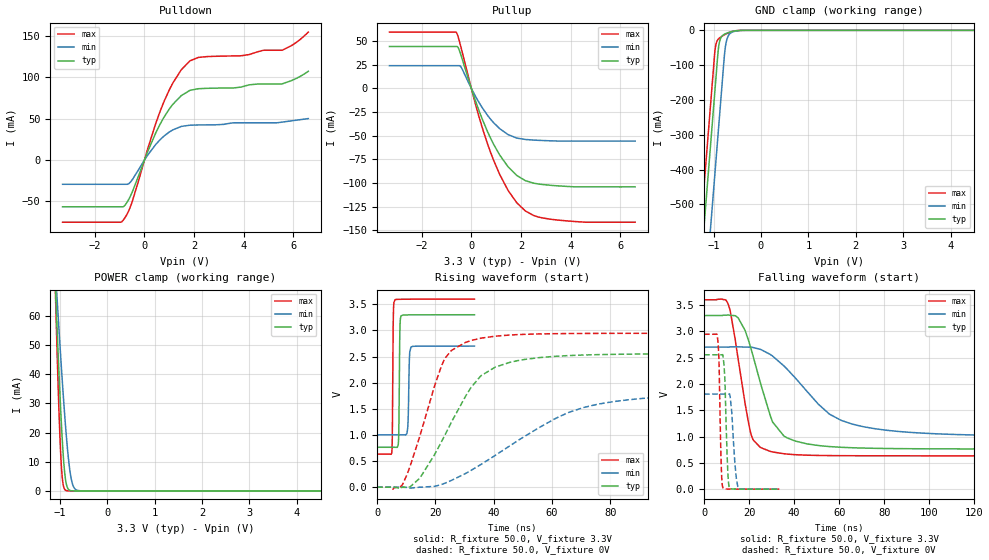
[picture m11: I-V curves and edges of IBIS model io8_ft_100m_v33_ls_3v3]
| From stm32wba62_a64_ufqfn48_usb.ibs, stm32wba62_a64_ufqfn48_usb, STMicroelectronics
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[Model]   io8_ft_100m_v33_ls_3v3
Model_type I/O
Polarity   Non-Inverting
Enable   Active-Low
| CAP_THRESHOLD on pad IOFT is "UDTCAPC" :
| Rising=30.0% of vddiom   Falling=70.0% of vddiom
| C_comp min and max val. don't necessarily correlate with the min and max pvt
| but are the smallest and greatest pad capacitance found.
| var   typ   min   max
C_comp   3.88673pF  3.77800pF  3.94187pF
|C_comp_pullup   2.41834pF  2.25933pF  2.53603pF
|C_comp_pulldown   1.46839pF  1.51868pF  1.40584pF
Vinl = 1.35V
Vinh = 1.8V
Vmeas = 1.65V   | Reference voltage for timing measurements
Cref  = 50.0pF   | Timing specification test load capacitance value
Rref  = 1.0MOhm   | Timing specification test load resistance value
Vref  = 1.815V   | Timing specification test load voltage
[Model Spec]
| TIME_THRESHOLD on pin ZIV33M is "CMOS" :
| Rising=50.0% of vddiom   Falling=50.0% of vddiom
Vinl 1.28450V 1.07450V 1.37050V
Vinh 1.79550V 1.51850V 1.89950V
| variable   typ   min   max
[Temperature Range] 25.0 140.0 -40.0
| variable   typ   min   max
[Voltage Range] 3.3V 2.7V 3.6V
| variable   typ   min   max
[POWER Clamp Reference] 3.3V 2.7V 3.6V
| variable   typ   min   max
[GND Clamp Reference] 0V 0V 0V
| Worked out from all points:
|   slope of the pulldown table from 0 to 0.495 V, typ, clamps not added: 14 ohm
|   slope of the pullup table from 0 to 0.495 V, typ, clamps not added: 13.8 ohm
|   GND clamp passes 1 mA (typ) near -0.51 V on its own axis
|   POWER clamp passes 1 mA (typ) near -0.83 V on its own axis
|   rising waveform, R_fixture 50.0, V_fixture 3.3V: 20-80 % time 263ps typ, 359ps min, 246ps max; typ from 0.764 V to 3.3 V
|   falling waveform, R_fixture 50.0, V_fixture 3.3V: 20-80 % time 10.6ns typ, 24.4ns min, 6.74ns max; typ from 3.3 V to 0.764 V
|   rising waveform, R_fixture 50.0, V_fixture 0V: 20-80 % time 15.8ns typ, 33.1ns min, 9.96ns max; typ from 0 V to 2.55 V
|   falling waveform, R_fixture 50.0, V_fixture 0V: 20-80 % time 1.09ns typ, 1.66ns min, 865ps max; typ from 2.55 V to 0 V
[POWER Clamp]
-3.3V     1.123A     753mA      1.645A
-1.09V    69.42mA    75.17mA    67.14mA
-1.08V    65.31mA    72.42mA    61.23mA
-1.06V    57.23mA    66.98mA    49.77mA
-1.01V    38.06mA    53.68mA    24.29mA
-970mV    24.36mA    43.46mA    9.575mA
-930mV    13.06mA    33.74mA    2.352mA
-870mV    3.065mA    20.56mA    165.9uA
-810mV    418.4uA    10.06mA    10.3uA
-760mV    69.41uA    4.321mA    1.009uA
-630mV    611.5nA    197uA      2.727nA
6.6V      0A         0A         0A
[GND Clamp]
-3.3V     -4.134A    -4.372A    -4.018A
-1.59V    -1.227A    -1.465A    -1.111A
-1.25V    -648.9mA   -886.9mA   -533mA
-980mV    -189.9mA   -427.9mA   -74mA
-960mV    -155.9mA   -393.9mA   -48.8mA
-910mV    -70.86mA   -308.9mA   -27.2mA
-880mV    -37.23mA   -257.9mA   -22.76mA
-770mV    -11.28mA   -71.59mA   -12.95mA
-730mV    -8.709mA   -32.74mA   -10.07mA
-630mV    -4.122mA   -6.943mA   -4.354mA
-370mV    -42.68uA   -212.2uA   -13.03uA
6.6V      2.31nA     506.4nA    1.057nA
| variable   typ   min   max
[Pullup Reference] 3.3V 2.7V 3.6V
| variable   typ   min   max
[Pulldown Reference] 0V 0V 0V
[Pullup]
-3.3V     44.29mA    24.03mA    59.52mA
-600mV    44.29mA    24.03mA    58.97mA
-520mV    42.47mA    24.03mA    53.36mA
-410mV    34.41mA    22.34mA    42.54mA
310mV     -23.64mA   -14.94mA   -30.17mA
890mV     -58.72mA   -36.07mA   -75.54mA
1.48V     -82.86mA   -48.82mA   -107.8mA
1.83V     -91.99mA   -52.47mA   -120.8mA
2.17V     -97.42mA   -53.93mA   -129.4mA
2.7V      -101mA     -54.85mA   -135.9mA
3.48V     -102.9mA   -55.62mA   -139.1mA
6.6V      -104.1mA   -55.62mA   -141.4mA
[Pulldown]
-3.3V     -56.7mA    -29.42mA   -75.36mA
-860mV    -56.67mA   -29.42mA   -72.94mA
-520mV    -40.69mA   -25.01mA   -52.64mA
460mV     33.25mA    19.09mA    44.92mA
800mV     52.54mA    29.36mA    71.75mA
1.14V     67.41mA    36.49mA    93.2mA
1.48V     77.97mA    40.67mA    109.3mA
1.83V     84.38mA    42.18mA    120.1mA
2.17V     86.37mA    42.45mA    124.3mA
3.88V     88.31mA    45.11mA    126.3mA
5.54V     92.28mA    45.89mA    133mA
6.6V      107.5mA    50.2mA     155mA
[Ramp]
dV/dt_r 1.53258V/15.4843ns 1.08428V/32.98714ns 1.76673V/9.86055ns
dV/dt_f 1.52157V/10.47685ns 1.01877V/24.02377ns 1.77971V/6.67032ns
R_load = 50.0
| Removed startup time: 0s 0s 0s  .
| Removed end time: 33.4ns.
[Rising Waveform]
R_fixture   = 50.0
V_fixture   = 3.3V
V_fixture_min = 2.7V
V_fixture_max = 3.6V
0s        764mV      1.002V     633.8mV
5ns       764.1mV    1.002V     653.2mV
5.55ns    764.1mV    1.002V     3.255V
6.15ns    764.1mV    1.002V     3.589V
7.35ns    913.7mV    1.002V     3.595V
7.8ns     2.993V     1.002V     3.595V
8.2ns     3.278V     1.002V     3.596V
10.5ns    3.297V     1.142V     3.597V
11.6ns    3.298V     2.684V     3.597V
33.4ns    3.3V       2.699V     3.6V
| Removed startup time: 0s 0s 0s  .
| Removed end time: 248.4ns.
[Falling Waveform]
R_fixture   = 50.0
V_fixture   = 3.3V
V_fixture_min = 2.7V
V_fixture_max = 3.6V
0s        3.3V       2.7V       3.6V
10.55ns   3.31V      2.7V       3.534V
11.75ns   3.303V     2.706V     3.362V
15.15ns   3.256V     2.706V     2.472V
20.95ns   2.656V     2.698V     1.032V
29.4ns    1.398V     2.561V     718.2mV
36.9ns    975.1mV    2.281V     666.7mV
55.6ns    809.9mV    1.429V     638.5mV
76.05ns   776.4mV    1.148V     634.6mV
248.4ns   764mV      1.002V     633.8mV
| Removed startup time: 0s 0s 0s  .
| Removed end time: 248.4ns.
[Rising Waveform]
R_fixture   = 50.0
V_fixture   = 0V
V_fixture_min = 0V
V_fixture_max = 0V
0s        20.88nV    123.8nV    58.45nV
8.45ns    -3.792mV   5.653uV    33.94mV
14.55ns   168mV      -370.6uV   957.9mV
19.8ns    633.7mV    18.35mV    1.953V
23.5ns    1.024V     82.11mV    2.481V
35.5ns    2.125V     430.3mV    2.85V
45.65ns   2.391V     795.8mV    2.912V
65.9ns    2.519V     1.434V     2.94V
86.2ns    2.546V     1.672V     2.944V
248.4ns   2.554V     1.807V     2.945V
| Removed startup time: 0s 0s 0s  .
| Removed end time: 33.4ns.
[Falling Waveform]
R_fixture   = 50.0
V_fixture   = 0V
V_fixture_min = 0V
V_fixture_max = 0V
0s        2.554V     1.807V     2.945V
6.15ns    2.554V     1.807V     2.823V
6.7ns     2.554V     1.807V     2.328V
7.65ns    2.554V     1.807V     439.3mV
8.35ns    2.551V     1.807V     31.17mV
9.2ns     2.132V     1.807V     5.295mV
10.25ns   636.4mV    1.807V     3.102mV
11.25ns   29.89mV    1.812V     2.891mV
15ns      1.775mV    46.24mV    784uV
33.4ns    226.6uV    441.1uV    142.7uV
